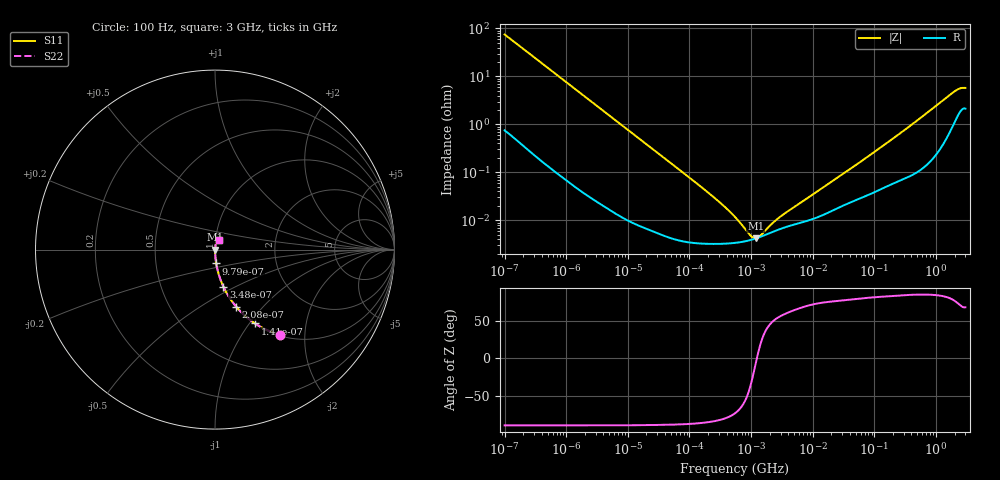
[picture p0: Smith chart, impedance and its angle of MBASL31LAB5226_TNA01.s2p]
! MBASL31LAB5226_TNA01  S-PARAMETER MODEL  ( Standard Model )
! Model Generated by TAIYO YUDEN Corporation (http://www.ty-top.com)
! Version 2.0
! TAIYO YUDEN Control No. 240725
! Copyright(c) 2012 TAIYO YUDEN CO.,LTD. All Rights Reserved.
! Product Description (link to TY-COMPAS)
! https://ds.yuden.co.jp/TYCOMPAS/or/detail?pn=MBASL31LAB5226KTNA01&u=M
! Products Name : Multilayer Ceramic Capacitors
! Characteristics :
!  Capacitance : 22 [uF] , Rated Voltage : 10 [V] , TCC : X5R
!  Case Size : 3.2 x 1.6 / 0.126 x 0.063 [mm/inch] , Thickness : 1.6 / 0.063 [mm/inch]
!  (Conditions: Temperature = 25 [degC] , DC Bias Voltage = 0 [V])
! External Node Assignments :
!  1  o---| |---o  2
! GND o---------o GND
! Frequency Range : 100Hz  -  3GHz  [ 401 STEP ]
# MHZ S RI R 50
! Freq[MHz].  S11 Real  S11 Imag  S21 Real  S21 Imag  S12 Real  S12 Imag  S22 Real  S22 Imag
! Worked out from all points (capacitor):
!   401 points, 100 Hz to 3 GHz, reference 50 ohm
!   read as one part in series: C = 21.2 uF near 109 Hz
!   lowest |Z| = 4.21 mohm at 1.189 MHz (marker M1)
!   series resonance near 1.238 MHz, so ESL is about 780 pH
!   S11 on the Smith chart (normalised r, x): 100 Hz: 1.02, -1.50; 141 Hz: 1.01, -1.07; 208 Hz: 1.01, -0.73; 348 Hz: 1.00, -0.43; 979 Hz: 1.00, -0.16; 3 GHz: 1.04, +0.11
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0.0001  0.3614 -0.4754  0.6386 0.4754  0.6386 0.4754  0.3614 -0.4754
0.000141  0.2235 -0.4117  0.7765 0.4117  0.7765 0.4117  0.2235 -0.4117
0.000208  0.1186 -0.3186  0.8814 0.3186  0.8814 0.3186  0.1186 -0.3186
0.000348  0.0467 -0.2065  0.9533 0.2065  0.9533 0.2065  0.0467 -0.2065
0.000559  0.0192 -0.1328  0.9808 0.1328  0.9808 0.1328  0.0192 -0.1328
0.000979  0.00668 -0.0771  0.9933 0.0771  0.9933 0.0771  0.00668 -0.0771
0.001788  0.00221 -0.0425  0.9978 0.0425  0.9978 0.0425  0.00221 -0.0425
0.005476  0.000351 -0.014  0.9996 0.014  0.9996 0.014  0.000351 -0.014
0.031977  5.82e-05 -0.00243  0.9999 0.00243  0.9999 0.00243  5.82e-05 -0.00243
0.221826  3.24e-05 -0.00034  1 0.00034  1 0.00034  3.24e-05 -0.00034
0.371814  3.26e-05 -0.00019  1 0.00019  1 0.00019  3.26e-05 -0.00019
0.547723  3.39e-05 -0.000113  1 0.000113  1 0.000113  3.39e-05 -0.000113
0.650627  3.49e-05 -8.49e-05  1 8.49e-05  1 8.49e-05  3.49e-05 -8.49e-05
1.188587  4.19e-05 -4.75e-06  1 4.75e-06  1 4.75e-06  4.19e-05 -4.75e-06
2.266852  5.77e-05 6.81e-05  0.9999 -6.81e-05  0.9999 -6.81e-05  5.77e-05 6.81e-05
2.579298  6.16e-05 8.26e-05  0.9999 -8.26e-05  0.9999 -8.26e-05  6.16e-05 8.26e-05
9.794414  0.000105 0.000322  0.9999 -0.000322  0.9999 -0.000322  0.000105 0.000322
52.48047  0.000271 0.00146  0.9997 -0.00146  0.9997 -0.00146  0.000271 0.00146
175.1444  0.000557 0.00444  0.9994 -0.00444  0.9994 -0.00444  0.000557 0.00444
1868.531  0.011 0.0441  0.989 -0.0441  0.989 -0.0441  0.011 0.0441
2419.119  0.02 0.0512  0.98 -0.0512  0.98 -0.0512  0.02 0.0512
3000  0.0236 0.0513  0.9764 -0.0513  0.9764 -0.0513  0.0236 0.0513
